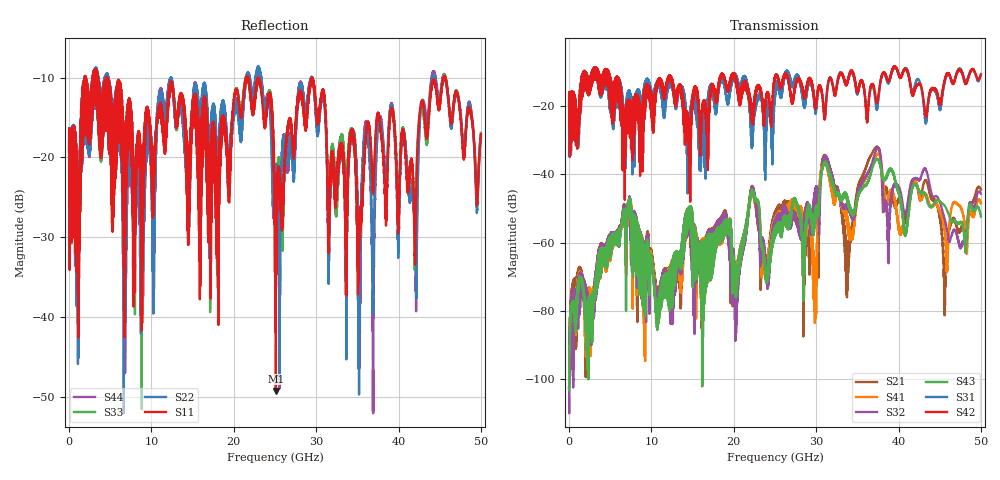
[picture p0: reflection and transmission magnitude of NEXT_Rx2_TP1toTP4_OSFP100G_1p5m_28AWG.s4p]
! Touchstone data
! Created: 27-Feb-2019 by IdEM 12 (12.1.0)
! COMMENTS
!  Created Wed Feb 27 09:43:39 2019
!  64 Port Network Data from SP1.SP block
!  freq  magS1_1  angS1_1  magS1_2  angS1_2  magS1_3  angS1_3  magS1_4  angS1_4
!  magS1_5  angS1_5  magS1_6  angS1_6  magS1_7  angS1_7  magS1_8  angS1_8
!  magS1_9  angS1_9  magS1_10  angS1_10  magS1_11  angS1_11  magS1_12  angS1_12
!  magS1_13  angS1_13  magS1_14  angS1_14  magS1_15  angS1_15  magS1_16  angS1_16
!  magS1_17  angS1_17  magS1_18  angS1_18  magS1_19  angS1_19  magS1_20  angS1_20
!  magS1_21  angS1_21  magS1_22  angS1_22  magS1_23  angS1_23  magS1_24  angS1_24
!  magS1_25  angS1_25  magS1_26  angS1_26  magS1_27  angS1_27  magS1_28  angS1_28
!  magS1_29  angS1_29  magS1_30  angS1_30  magS1_31  angS1_31  magS1_32  angS1_32
!  magS1_33  angS1_33  magS1_34  angS1_34  magS1_35  angS1_35  magS1_36  angS1_36
!  magS1_37  angS1_37  magS1_38  angS1_38  magS1_39  angS1_39  magS1_40  angS1_40
!  magS1_41  angS1_41  magS1_42  angS1_42  magS1_43  angS1_43  magS1_44  angS1_44
!  magS1_45  angS1_45  magS1_46  angS1_46  magS1_47  angS1_47  magS1_48  angS1_48
!  magS1_49  angS1_49  magS1_50  angS1_50  magS1_51  angS1_51  magS1_52  angS1_52
!  magS1_53  angS1_53  magS1_54  angS1_54  magS1_55  angS1_55  magS1_56  angS1_56
!  magS1_57  angS1_57  magS1_58  angS1_58  magS1_59  angS1_59  magS1_60  angS1_60
!  magS1_61  angS1_61  magS1_62  angS1_62  magS1_63  angS1_63  magS1_64  angS1_64
!  magS2_1  angS2_1  magS2_2  angS2_2  magS2_3  angS2_3  magS2_4  angS2_4
!  magS2_5  angS2_5  magS2_6  angS2_6  magS2_7  angS2_7  magS2_8  angS2_8
!  magS2_9  angS2_9  magS2_10  angS2_10  magS2_11  angS2_11  magS2_12  angS2_12
!  magS2_13  angS2_13  magS2_14  angS2_14  magS2_15  angS2_15  magS2_16  angS2_16
!  magS2_17  angS2_17  magS2_18  angS2_18  magS2_19  angS2_19  magS2_20  angS2_20
!  magS2_21  angS2_21  magS2_22  angS2_22  magS2_23  angS2_23  magS2_24  angS2_24
!  magS2_25  angS2_25  magS2_26  angS2_26  magS2_27  angS2_27  magS2_28  angS2_28
!  magS2_29  angS2_29  magS2_30  angS2_30  magS2_31  angS2_31  magS2_32  angS2_32
!  magS2_33  angS2_33  magS2_34  angS2_34  magS2_35  angS2_35  magS2_36  angS2_36
!  magS2_37  angS2_37  magS2_38  angS2_38  magS2_39  angS2_39  magS2_40  angS2_40
!  magS2_41  angS2_41  magS2_42  angS2_42  magS2_43  angS2_43  magS2_44  angS2_44
!  magS2_45  angS2_45  magS2_46  angS2_46  magS2_47  angS2_47  magS2_48  angS2_48
!  magS2_49  angS2_49  magS2_50  angS2_50  magS2_51  angS2_51  magS2_52  angS2_52
!  magS2_53  angS2_53  magS2_54  angS2_54  magS2_55  angS2_55  magS2_56  angS2_56
!  magS2_57  angS2_57  magS2_58  angS2_58  magS2_59  angS2_59  magS2_60  angS2_60
!  magS2_61  angS2_61  magS2_62  angS2_62  magS2_63  angS2_63  magS2_64  angS2_64
!  magS3_1  angS3_1  magS3_2  angS3_2  magS3_3  angS3_3  magS3_4  angS3_4
!  magS3_5  angS3_5  magS3_6  angS3_6  magS3_7  angS3_7  magS3_8  angS3_8
!  magS3_9  angS3_9  magS3_10  angS3_10  magS3_11  angS3_11  magS3_12  angS3_12
!  magS3_13  angS3_13  magS3_14  angS3_14  magS3_15  angS3_15  magS3_16  angS3_16
!  magS3_17  angS3_17  magS3_18  angS3_18  magS3_19  angS3_19  magS3_20  angS3_20
!  magS3_21  angS3_21  magS3_22  angS3_22  magS3_23  angS3_23  magS3_24  angS3_24
!  magS3_25  angS3_25  magS3_26  angS3_26  magS3_27  angS3_27  magS3_28  angS3_28
!  magS3_29  angS3_29  magS3_30  angS3_30  magS3_31  angS3_31  magS3_32  angS3_32
!  magS3_33  angS3_33  magS3_34  angS3_34  magS3_35  angS3_35  magS3_36  angS3_36
!  magS3_37  angS3_37  magS3_38  angS3_38  magS3_39  angS3_39  magS3_40  angS3_40
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# Hz S MA R 50
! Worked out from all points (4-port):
!   5000 points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, 10 MHz to 50 GHz, reference 50 ohm
!   strongest paths, dB at 10 MHz, 12.51 GHz, 25.01 GHz, 37.51 GHz, 50 GHz:
!     S42: -19.6, -12.4, -11.6, -17.8, -10.7
!     S31: -19.6, -14.0, -15.9, -19.1, -11.0
!     S43: -103.2, -79.2, -57.4, -35.6, -52.3
!     S32: -105.5, -80.3, -55.7, -32.3, -45.6
!     S41: -102.7, -76.0, -54.2, -34.0, -48.5
!     S21: -102.4, -76.6, -52.8, -32.0, -44.4
!   lowest |S11| = -49.2 dB at 25.11 GHz (marker M1), VSWR 1.01, Z = 50.3 + j0.113 ohm
!   |S11| at or under -10 dB: 4.66 GHz to 21.51 GHz (16.85 GHz wide, 129 % of centre); 22.94 GHz to 45.47 GHz (22.53 GHz wide, 65.9 % of centre); 45.68 GHz to end of sweep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
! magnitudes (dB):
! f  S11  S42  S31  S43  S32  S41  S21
! 10 MHz  -19.2  -19.6  -19.6  -103.2  -105.5  -102.7  -102.4
! 7.27 GHz  -12.6  -18.2  -15.3  -48.4  -47.5  -49.8  -49.1
! 10.71 GHz  -15.1  -14.3  -12.9  -85.6  -79.1  -77.3  -75.4
! 25.11 GHz  -49.2  -11.2  -14.8  -57.1  -55.2  -53.9  -52.3
! 37.38 GHz  -14.9  -18.9  -20.6  -35.4  -32.5  -34.1  -31.9
! 45.64 GHz  -10.0  -11.8  -12.4  -49.3  -53.5  -57.4  -78.5
! 50 GHz  -17.1  -10.7  -11.0  -52.3  -45.6  -48.5  -44.4
